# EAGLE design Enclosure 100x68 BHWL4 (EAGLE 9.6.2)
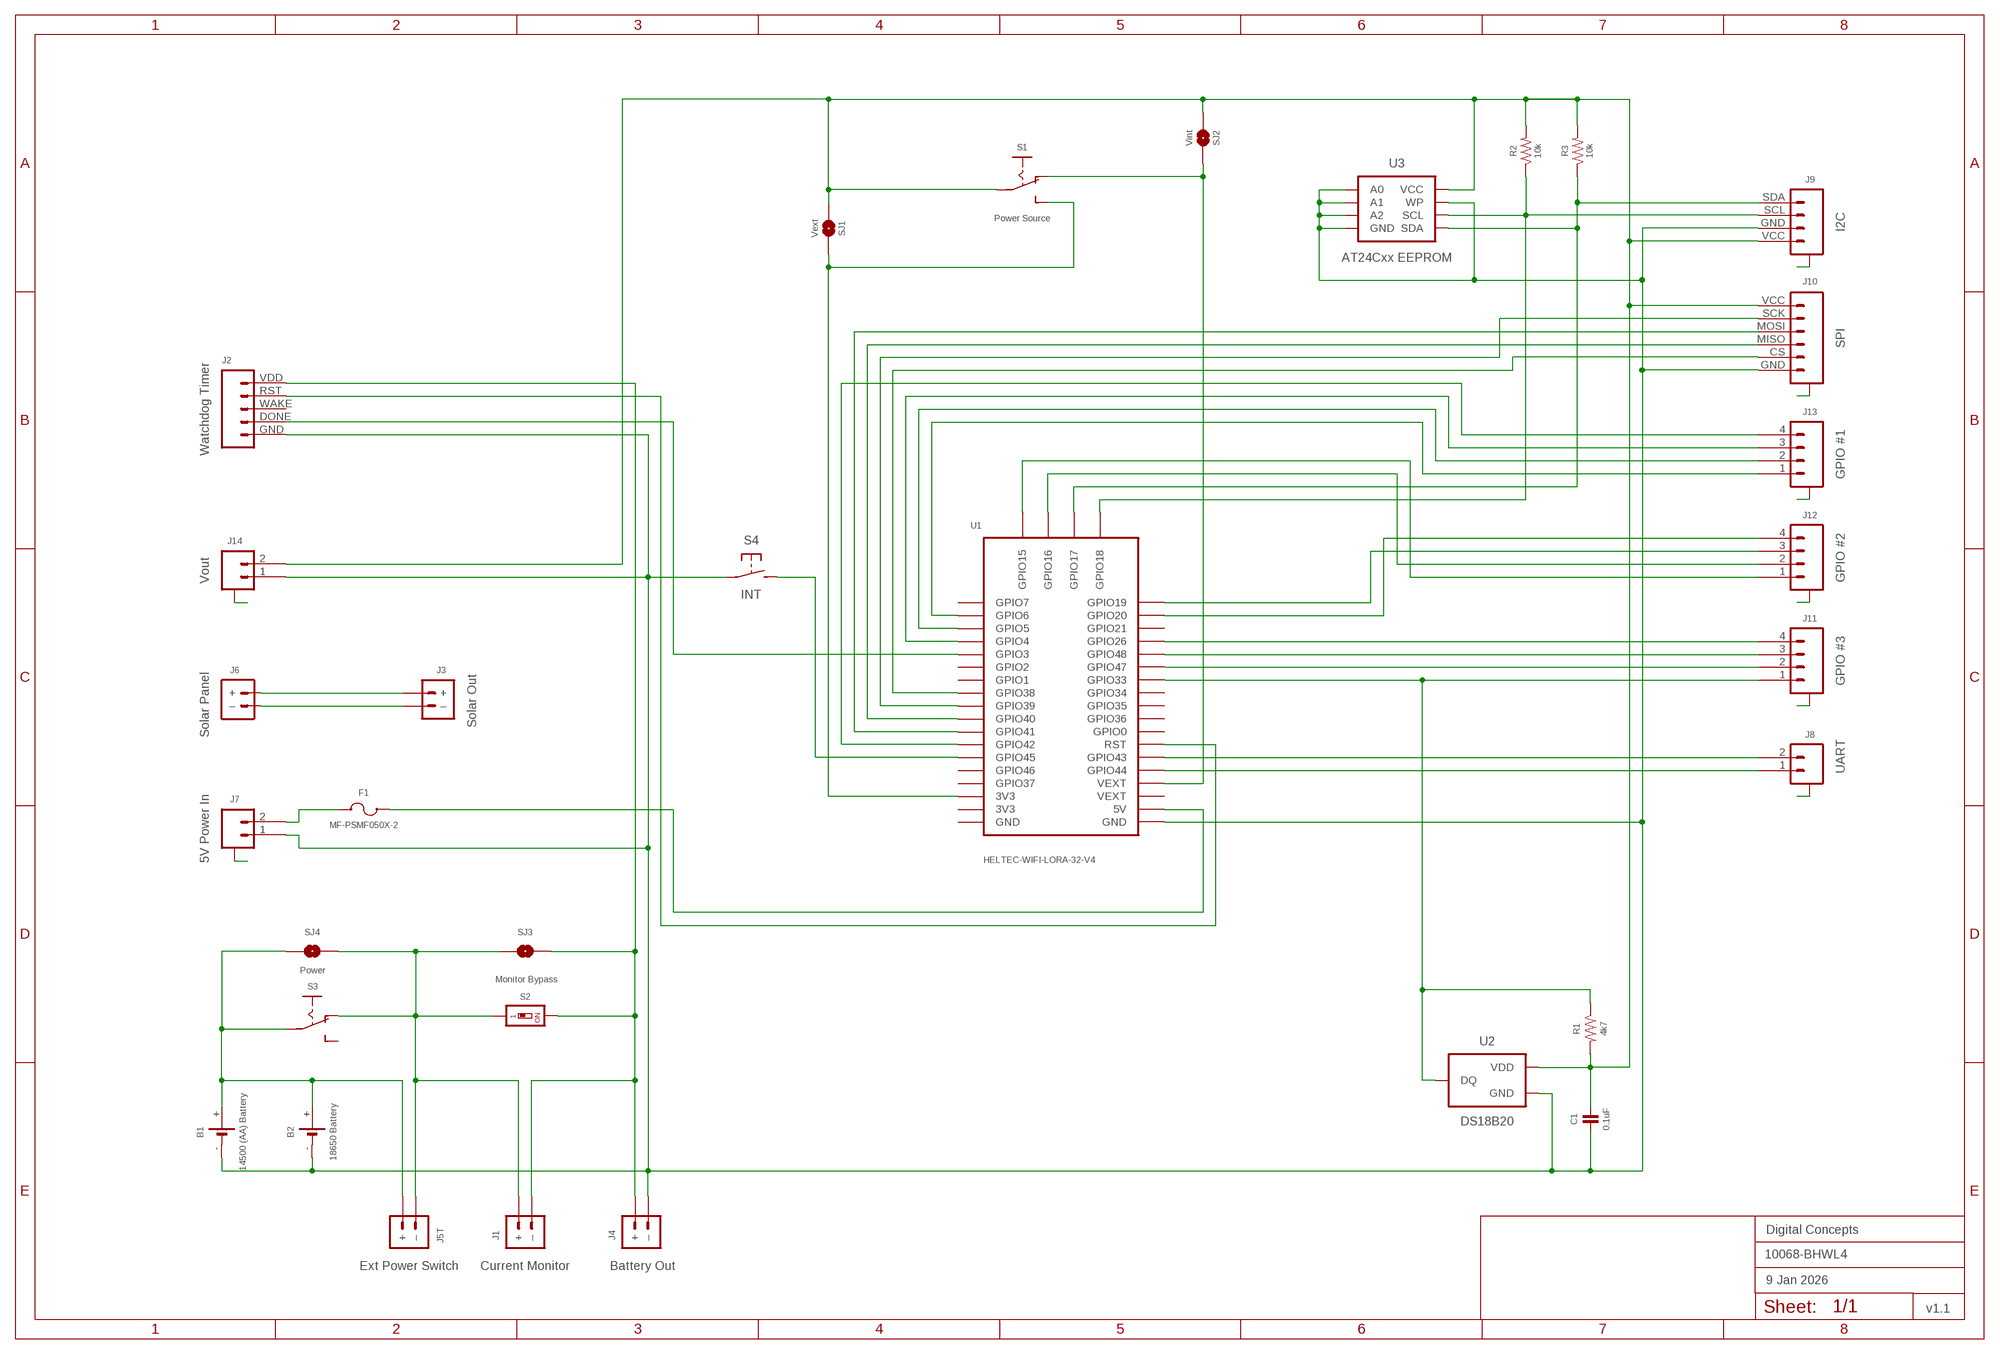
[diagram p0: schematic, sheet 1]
FRAME2 (A3L-LOC): DATE: 9 Jan 2026; OWNER: Digital Concepts; TITLE: 10068-BHWL4; VERSION: v1.1

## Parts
B1  14500 (AA) Battery  BATTERY-HOLDER-14500(AA)  [BATTERY-14500]
B2  18650 Battery  BATTERY-HOLDER-18650  [BATTERY-18650]
C1  0.1uF  CAPACITOR-0805  [C0805]
F1  MF-PSMF050X-2  [F0805]
J1  Current Monitor  JST-PH2.0-2-HORIZONTALJST-PTH-2  [JST-PH2.0-2-HORIZONTAL]
J2  Watchdog Timer  HEADER-1X5-WDT  [CONN_05-WDT]
J3  Solar Out  JST-GH1.25-2-HORIZONTAL-POWER  [JST-GH1.25-2-HORIZONTAL]
J4  Battery Out  JST-GH1.25-2-HORIZONTAL-POWER  [JST-GH1.25-2-HORIZONTAL]
J5T  Ext Power Switch  JST-PH2.0-2-DUAL-POWERJST-PTH-2  [JST-PH2.0-2-DUAL-POWER]
J6  Solar Panel  JST-PH2.0-2-VERTICAL  [JST-PH2.0-2-VERTICAL=POWER]
J7  5V Power In  JST-SH1.0-2-SMD-HORIZONTAL  [JST-SH1.0-2-SMD-HORIZONTAL]
J8  UART  JST-SH1.0-2-SMD-HORIZONTAL  [JST-SH1.0-2-SMD-HORIZONTAL]
J9  I2C  JST-SH1.0-4-SMD-HORIZONTAL-I2C  [JST-SH1.0-4-SMD-HORIZONTAL-I2C]
J10  SPI  JST-SH1.0-6-SMD-HORIZONTAL-SPI  [JST-SH1.0-6-SMD-HORIZONTAL-SPI]
J11  GPIO #3  JST-SH1.0-4-SMD-HORIZONTAL  [JST-SH1.0-4-SMD-HORIZONTAL]
J12  GPIO #2  JST-SH1.0-4-SMD-HORIZONTAL  [JST-SH1.0-4-SMD-HORIZONTAL]
J13  GPIO #1  JST-SH1.0-4-SMD-HORIZONTAL  [JST-SH1.0-4-SMD-HORIZONTAL]
J14  Vout  JST-SH1.0-2-SMD-HORIZONTAL  [JST-SH1.0-2-SMD-HORIZONTAL]
R1  4k7  RESISTORR0805  [R0805]
R2  10k  RESISTORR0805  [R0805]
R3  10k  RESISTORR0805  [R0805]
S1  Power Source  SWITCH-SLIDE-SPDT-SMT  [SWITCH-SPDT-SMT]
S2  Monitor Bypass  SWITCH-DIP-SWS001  [SMD-001]
S3  Power  SWITCH-SLIDE-SPDT-PTH  [SWITCH-SPDT-PTH]
S4  INT  SWITCH-MOMENTARY-2-PIN  [SWITCH-2-PAD]
SJ1  Vext  SJ  [SJ]
SJ2  Vint  SJ-V-2  [SJ-VIA-2]
SJ3  Monitor  SJ  [SJ]
SJ4  Power  SJ  [SJ]
U1  HELTEC-WIFI-LORA-32-V4  [HELTEC-WIFI-LORA-32-V4]
U2  DS18B20  THERMOMETER-DS18B20  [TO-92]
U3  AT24Cxx EEPROM  AT24CXX-EEPROM  [SOP-8]

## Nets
3V3: S1.3(S) SJ1.1 U1.3V3@38(3V3)
5V: F1.1 U1.5V
A2: J11.A@1(A) J11.A@4(A)
A3: J12.A@1(A) J12.A@4(A)
A4: J10.A@1(A) J10.A@6(A)
A5: J14.A@1(A) J14.A@2(A)
A6: J8.A@1(A) J8.A@2(A)
A7: J9.A@1(A) J9.A@4(A)
A8: J13.A@1(A) J13.A@4(A)
A13: J7.A@1(A) J7.A@2(A)
BAT+: B1.+ B2.+ J5T.+ S3.2(P) SJ4.2
CS: J10.CS U1.GPIO38
GND: B1.- B2.- C1.2 J2.GND J4.-(–) J7.1 J9.GND J10.GND J14.1 S4.P$1(P) U1.GND@1(GND) U2.1(GND) U3.P$1(A0) U3.P$2(A1) U3.P$3(A2) U3.P$4(GND) U3.P$7(WP)
GPIO3: J2.DONE U1.GPIO3
GPIO4: J13.3 U1.GPIO4
GPIO5: J13.2 U1.GPIO5
GPIO6: J13.1 U1.GPIO6
GPIO15: J12.1 U1.GPIO15
GPIO16: J12.2 U1.GPIO16
GPIO19: J12.3 U1.GPIO19
GPIO20: J12.4 U1.GPIO20
GPIO26: J11.4 U1.GPIO26
GPIO33: J11.1 R1.1 U1.GPIO33 U2.2(DQ)
GPIO42: J13.4 U1.GPIO42
GPIO45: S4.P$2(S) U1.GPIO45
GPIO47: J11.2 U1.GPIO47
GPIO48: J11.3 U1.GPIO48
MCU-BAT+: J1.2(–) J2.VDD J4.+ S2.2 SJ3.1
MISO: J10.MISO U1.GPIO40
MOSI: J10.MOSI U1.GPIO41
N$14: F1.2 J7.2
POWER+: J1.1(+) J5T.-(–) S2.1 S3.1(O) SJ3.2 SJ4.1
RST: J2.RST U1.RST
RX: J8.1 U1.GPIO44
SCK: J10.SCK U1.GPIO39
SCL: J9.SCL R2.1 U1.GPIO18 U3.P$6(SCL)
SDA: J9.SDA R3.1 U1.GPIO17 U3.P$5(SDA)
SOLAR+: J3.+ J6.+
SOLAR-: J3.-(–) J6.-(–)
TX: J8.2 U1.GPIO43
VCC: C1.1 J9.VCC J10.VCC J14.2 R1.2 R2.2 R3.2 S1.2(P) SJ1.2 SJ2.2 SJ2.2@V U2.3(VDD) U3.P$8(VCC)
VEXT: S1.1(O) SJ2.1 U1.VEXT@4(VEXT)
Unconnected: J2.WAKE S3.3(S) U1.3V3@39(3V3) U1.GND@40(GND) U1.GPIO0 U1.GPIO1 U1.GPIO2 U1.GPIO7 U1.GPIO21 U1.GPIO34 U1.GPIO35 U1.GPIO36 U1.GPIO37 U1.GPIO46 U1.VEXT@3(VEXT)

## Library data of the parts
B1 = digitalconcepts:BATTERY-HOLDER-14500(AA): 14500 (AA) battery holder
B2 = digitalconcepts:BATTERY-HOLDER-18650: 18650 Battery Holder
C1 = digitalconcepts:CAPACITOR-0805: 0805 Capacitor
F1 = digitalconcepts:MF-PSMF050X-2: PTC Resettable Fuse
J1 = digitalconcepts:JST-PH2.0-2-HORIZONTAL: PH2.0 2P Right Angle PCB Connector; PROD_ID: CONN-09863; SKU: PRT-09914
J2 = digitalconcepts:HEADER-1X5-WDT: Single Row 5-Pin Header
J3 J4 = digitalconcepts:JST-GH1.25-2-HORIZONTAL-POWER: JST GH1.25 2P PTH Connector (Power)
J5T = digitalconcepts:JST-PH2.0-2-DUAL-POWER: JST PH2.0 2P PTH Dual-Side Connector (Power); PROD_ID: CONN-09863; SKU: PRT-09914
J6 = digitalconcepts:JST-PH2.0-2-VERTICAL: PH2.0 2P PCB Connector
J7 J8 J14 = digitalconcepts:JST-SH1.0-2-SMD-HORIZONTAL: JST SH1.0 2P SMD Horizontal Connector
J9 = digitalconcepts:JST-SH1.0-4-SMD-HORIZONTAL-I2C: JST SH1.0 4P SMD I2C horizontal connector
J10 = digitalconcepts:JST-SH1.0-6-SMD-HORIZONTAL-SPI: JST SH1.0 6P SMD SPI horizontal connector
J11-J13 = digitalconcepts:JST-SH1.0-4-SMD-HORIZONTAL: JST SH1.0 4P SMD horizontal connector
R1-R3 = digitalconcepts:RESISTOR: Resistor; SPICEPREFIX: R
S1 = digitalconcepts:SWITCH-SLIDE-SPDT-SMT: Mini Sliding Switch SPDT SMT
S2 = digitalconcepts:SWITCH-DIP-SWS001: SMD Dip Switch 1 pol.
S3 = digitalconcepts:SWITCH-SLIDE-SPDT-PTH: Mini Sliding Switch SPDT PTH
S4 = digitalconcepts:SWITCH-MOMENTARY-2-PIN: 2 Pin Momentary Switch
SJ1 SJ3 SJ4 = digitalconcepts:SJ: Solder Jumper
SJ2 = digitalconcepts:SJ-V-2: Solder Jumper with Pad Vias
U1 = digitalconcepts:HELTEC-WIFI-LORA-32-V4: Heltec WiFi LoRa 32 Development Board V4
U2 = digitalconcepts:THERMOMETER-DS18B20: Digital Thermometer -55C-125C TO92-3; AVAILABILITY: Bad; DESCRIPTION: Temperature Sensor Digital, Local -55°C ~ 125°C 12 b 8-uMAX; MF: Maxim Integrated; MP: DS18B20; PACKAGE: TO-92 Maxim Integrated; PRICE: None
U3 = digitalconcepts:AT24CXX-EEPROM: AT24Cxx EEPROM SOP-8

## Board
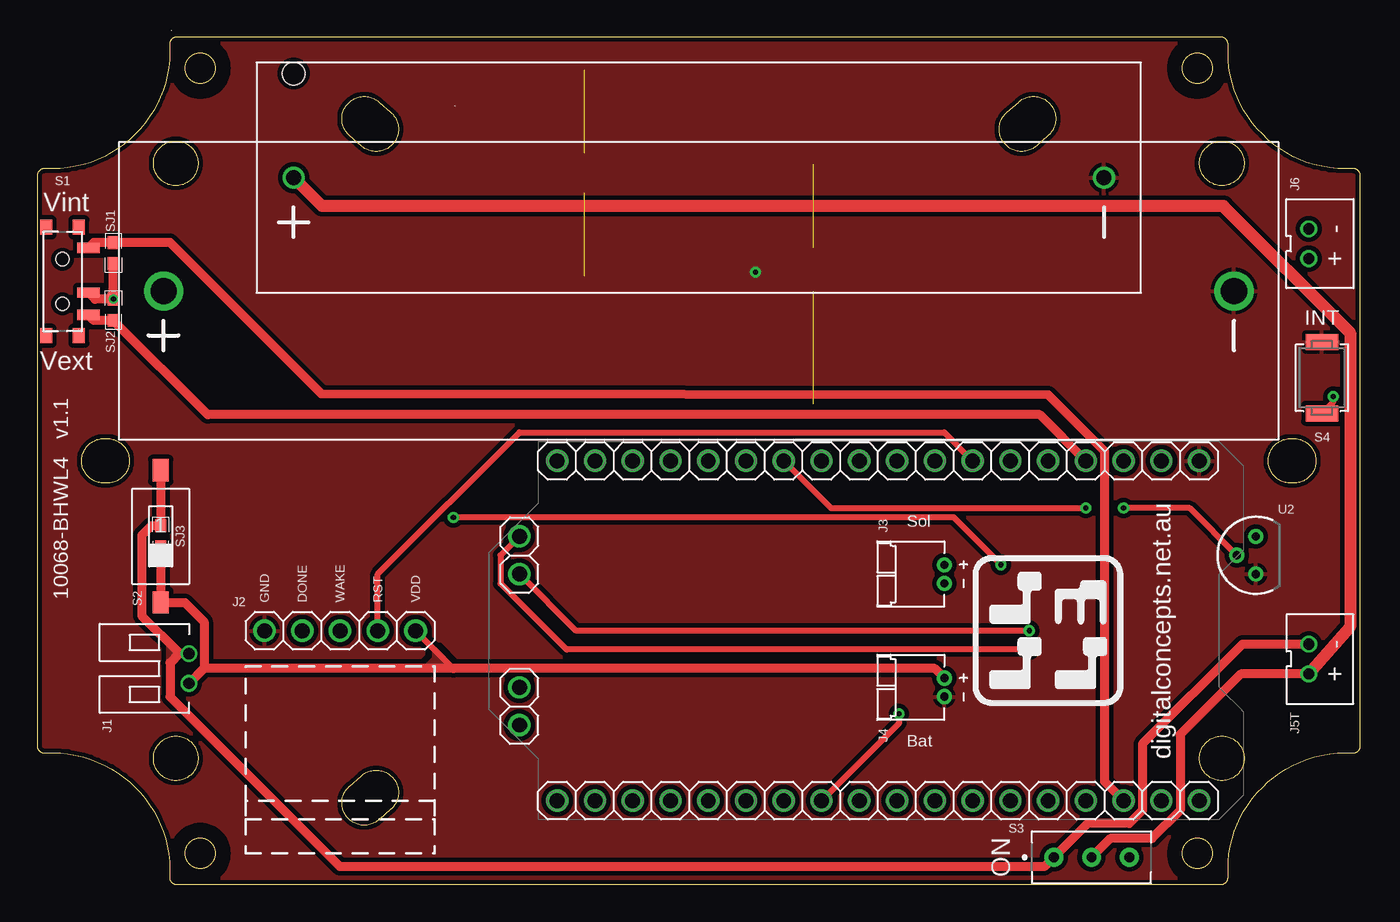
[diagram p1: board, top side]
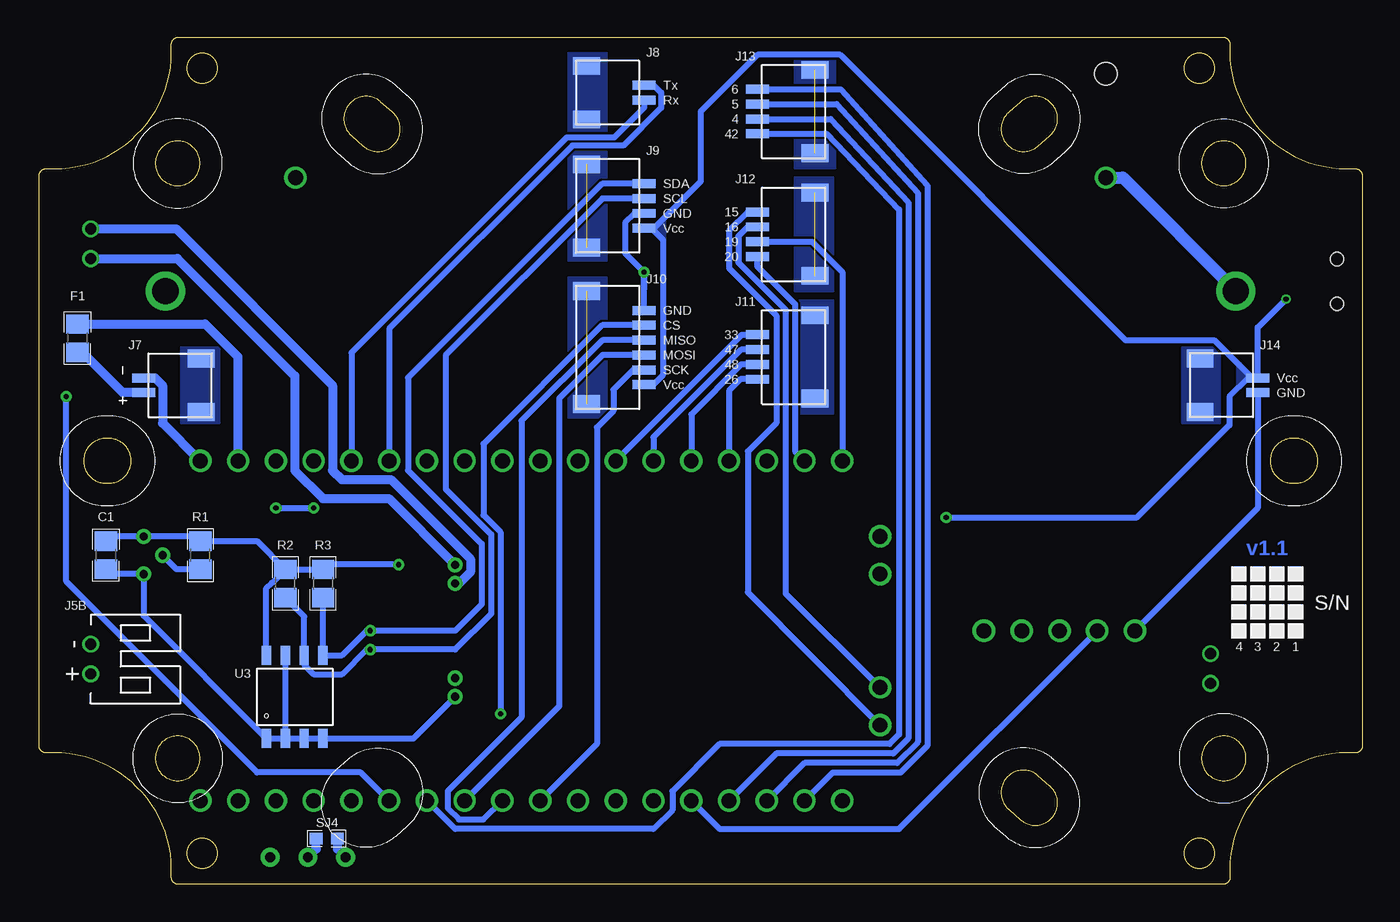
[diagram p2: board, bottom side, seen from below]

Size 89 x 57 mm. Coordinates in mm from the lower left corner, seen from the top.
Outline: 1134 segments
Outline: circle at 10.97,2.08 radius 1.02
Outline: circle at 10.97,54.92 radius 1.02
Outline: circle at 78.03,54.92 radius 1.02
Outline: circle at 78.03,2.08 radius 1.02
Copper layers (1*16): Top 0.035mm / dielectric 1.5mm / Bottom 0.035mm
Design rules "default *": minimum track width 6mil, minimum drill 0.35mm, track to track 6mil, track to pad 6mil, pad to pad 6mil, via to via 6mil, smd to smd 6mil, copper to edge 6mil, drill to drill 6mil, minimum pad ring 1mil, minimum via ring 8mil, stop-mask expansion 4mil, vias tented up to drill 0mil, thermal gap 10mil

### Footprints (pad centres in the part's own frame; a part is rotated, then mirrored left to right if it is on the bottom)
BATTERY-14500 = drill 1: + -27.25,0; - 27.25,0 | hole 1.524: -27.25,7
BATTERY-18650 = drill 1.75: + -36,0; - 36,0
C0805 = smd 1.3 x 1.5: 1 -0.95,0; 2 0.95,0
F0805 = smd 1.3 x 1.5: 1 -0.95,0; 2 0.95,0
JST-PH2.0-2-HORIZONTAL = drill 0.75: 1 1,0; 2 -1,0
CONN_05-WDT = drill 1 pad 1.524: DONE 2.54,0; GND 0,0; RST 7.62,0; VDD 10.16,0; WAKE 5.08,0
JST-GH1.25-2-HORIZONTAL = drill 0.55 pad 1.016: + -0.625,0; - 0.625,0
JST-PH2.0-2-DUAL-POWER = drill 0.75: + 1,0; - -1,0
JST-PH2.0-2-VERTICAL=POWER = drill 0.75: + -1,0; - 1,0
JST-SH1.0-2-SMD-HORIZONTAL = smd 0.6 x 1.55: 1 0.5,2.54; 2 -0.5,2.54 | smd 1.2 x 1.8: A@1 1.8,-1.335; A@2 -1.8,-1.335
JST-SH1.0-4-SMD-HORIZONTAL-I2C = smd 1.2 x 1.8: A@1 2.8,-1.335; A@4 -2.8,-1.335 | smd 0.6 x 1.55: GND 0.5,2.54; SCL -0.5,2.54; SDA -1.5,2.54; VCC 1.5,2.54
JST-SH1.0-6-SMD-HORIZONTAL-SPI = smd 1.2 x 1.8: A@1 3.8,-1.335; A@6 -3.8,-1.335 | smd 0.6 x 1.55: CS -1.5,2.54; GND -2.5,2.54; MISO -0.5,2.54; MOSI 0.5,2.54; SCK 1.5,2.54; VCC 2.5,2.54
JST-SH1.0-4-SMD-HORIZONTAL = smd 0.6 x 1.55: 1 1.5,2.54; 2 0.5,2.54; 3 -0.5,2.54; 4 -1.5,2.54 | smd 1.2 x 1.8: A@1 2.8,-1.335; A@4 -2.8,-1.335
R0805 = smd 1.3 x 1.5: 1 -0.95,0; 2 0.95,0
SWITCH-SPDT-SMT = smd 0.7 x 1.5: 1 2.25,1.75; 2 0.75,1.75; 3 -2.25,1.75 | smd 1 x 0.8: GND@1 3.65,-1.1; GND@2 3.65,1.1; GND@3 -3.65,1.1; GND@4 -3.65,-1.1 | hole 0.9: -1.5,0; 1.5,0
SMD-001 = smd 1.1 x 1.5: 1 0,-4.45; 2 0,4.45
SWITCH-SPDT-PTH = drill 0.65 pad 1.27: 1 -2.54,0; 2 0,0; 3 2.54,0
SWITCH-2-PAD = smd 1.067 x 2.184: P$1 -2.4,0; P$2 2.4,0
SJ = smd 0.864 x 0.762: 1 -0.711,0; 2 0.711,0
SJ-VIA-2 = smd 0.864 x 0.762: 1 -0.711,0; 2 0.711,0 | drill 0.35 pad 0.61: 2@V 0.711,0
HELTEC-WIFI-LORA-32-V4 = drill 1: 3V3@38 -22.86,5.08; 3V3@39 -22.86,2.54; 5V 0,2.54; GND@1 0,0; GND@40 -22.86,0; GPIO0 0,17.78; GPIO1 -22.86,27.94; GPIO2 -22.86,30.48; GPIO3 -22.86,33.02; GPIO4 -22.86,35.56; GPIO5 -22.86,38.1; GPIO6 -22.86,40.64; GPIO7 -22.86,43.18; GPIO15 -17.78,45.72; GPIO16 -15.24,45.72; GPIO17 -7.62,45.72; GPIO18 -5.08,45.72; GPIO19 0,43.18; GPIO20 0,40.64; GPIO21 0,38.1; GPIO26 0,35.56; GPIO33 0,27.94; GPIO34 0,25.4; GPIO35 0,22.86; GPIO36 0,20.32; GPIO37 -22.86,7.62; GPIO38 -22.86,25.4; GPIO39 -22.86,22.86; GPIO40 -22.86,20.32; GPIO41 -22.86,17.78; GPIO42 -22.86,15.24; GPIO43 0,12.7; GPIO44 0,10.16; GPIO45 -22.86,12.7; GPIO46 -22.86,10.16; GPIO47 0,30.48; GPIO48 0,33.02; RST 0,15.24; VEXT@3 0,5.08; VEXT@4 0,7.62
TO-92 = drill 0.55 pad 1.016: 1 -1.27,0; 2 0,1.27; 3 1.27,0
SOP-8 = smd 0.635 x 1.27: P$1 -1.905,-2.794; P$2 -0.635,-2.794; P$3 0.635,-2.794; P$4 1.905,-2.794; P$5 1.905,2.794; P$6 0.635,2.794; P$7 -0.635,2.794; P$8 -1.905,2.794

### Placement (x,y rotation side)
B1  44.5,47.55 0 top
B2  44.5,39.93 0 top
C1  84.5,22.15 270 bottom
F1  86.41,36.75 270 bottom
J1  10.21,14.53 90 top
J2  15.29,17.07 0 top
J3  61.01,20.88 270 top
J4  61.01,13.26 270 top
J5T  85.52,15.16 270 bottom
J6  85.52,43.1 90 top
J7  79.42,33.58 90 bottom
J8  50.85,53.26 270 bottom
J9  50.85,45.64 270 bottom
J10  50.85,36.12 270 bottom
J11  38.15,35.48 90 bottom
J12  38.15,43.74 90 bottom
J13  38.15,51.99 90 bottom
J14  9.57,33.58 270 bottom
R1  78.15,22.15 90 bottom
R2  72.44,20.24 90 bottom
R3  69.9,20.24 90 bottom
S1  1.7,40.56 270 top
S2  8.3,23.42 180 top
S3  70.92,1.83 0 top
S4  86.41,34.09 270 top
SJ1  5.13,42.47 270 top
SJ2  5.13,38.66 90 top
SJ3  8.3,23.42 90 top
SJ4  69.65,3.1 180 bottom
U1  78.15,28.5 90 top
U2  81.96,22.15 90 top
U3  71.8,12.62 0 bottom

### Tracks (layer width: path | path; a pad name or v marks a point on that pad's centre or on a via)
3V3
  Top 0.61: S1.3 3.82,43.18 SJ1.1 8.94,43.18 19.12,33 68,32.94 71.8,29.13 71.8,6.91 U1.3V3@38
5V
  Bottom 0.61: F1.1 77.83,37.7 75.61,35.48 U1.5V
$X
  cutout Bottom: 10.97,56.95 arc180 10.97,52.88 arc180
$X1
  cutout Bottom: 78.03,56.95 arc180 78.03,52.88 arc180
$X2
  cutout Top: 78.03,4.12 arc180 78.03,0.05 arc180
$X3
  cutout Top: 10.97,4.12 arc180 10.97,0.05 arc180
$X4
  cutout Top: 10.97,56.95 arc180 10.97,52.88 arc180
$X5
  cutout Top: 78.03,56.95 arc180 78.03,52.88 arc180
$X6
  cutout Bottom: 78.03,4.12 arc180 78.03,0.05 arc180
$X7
  cutout Bottom: 10.97,4.12 arc180 10.97,0.05 arc180
A2
  pour Bottom (no thermals): 35.61,39.29 38.15,39.29 38.15,31.67 35.61,31.67
A3  (1 unrouted)
  pour Bottom (no thermals): 35.61,47.55 38.15,47.55 38.15,39.93 35.61,39.93
A4  (1 unrouted)
  pour Bottom (no thermals): 50.85,31.42 53.39,31.42 53.39,40.82 50.85,40.82
A5
  pour Bottom (no thermals): 9.57,36.12 12.11,36.12 12.11,31.04 9.57,31.04
A6
  pour Bottom (no thermals): 53.39,55.93 53.39,50.6 50.85,50.6 50.85,55.93
A7  (1 unrouted)
  pour Bottom (no thermals): 50.85,49.33 53.39,49.33 53.39,41.96 50.85,41.96
A8  (1 unrouted)
  pour Bottom (no thermals): 35.48,55.8 38.15,55.8 38.15,48.18 35.48,48.18
A13
  pour Bottom (no thermals): 79.42,36.12 76.88,36.12 76.88,31.04 79.42,31.04
BAT+
  Top 0.61: J5T.+ 80.96,14.16 76.88,10.08 76.88,5 74.98,3.1 72.19,3.1 S3.2
  Top 0.813: B1.+ 19.15,45.64 79.79,45.64 88.31,37.12 88.31,17.34 J5T.+
  Bottom 0.61: S3.2 70.36,2.39 SJ4.2
  Bottom 0.813: B1.+ 16.12,47.55 B2.+
CS  (via drill 0.35)
  Top 0.406: v57.96,11.48 57.96,10.85 U1.GPIO38
  Bottom 0.406: J10.CS 51.13,37.62 59.1,29.64 59.1,24.84 57.96,23.7 v57.96,11.48
GND  (via drill 0.35)
  Bottom 0.406: U3.P$7 U3.P$2 | U3.P$2 U3.P$1 81.96,18.09 U2.1 84.42,20.88 C1.2 | U3.P$2 U3.P$3 U3.P$4 63.81,9.83 J4.- | J10.GND v48.31,41.2 | v48.31,41.2 48.31,40.06 | J9.GND 48.94,45.14 49.58,44.51 49.58,42.47 v48.31,41.2 | J2.GND 7.03,25.32 J14.1
  Bottom 0.61: U1.GND@1 80.69,31.04 80.69,33.57 81.2,34.08 J7.1
  pour Top (isolate 0.305, rank 2): -1.65,58.87 -1.65,-1.92 90.59,-1.92 90.59,58.87
GPIO3
  Bottom 0.406: J2.DONE 31.16,3.73 43.23,3.73 U1.GPIO3
GPIO4
  Bottom 0.406: J13.3 35.74,51.49 30.53,45.9 30.53,9.83 31.55,8.81 39.42,8.81 U1.GPIO4
GPIO5
  Bottom 0.406: J13.2 35.35,52.49 29.89,46.53 29.89,9.58 31.29,8.18 37.51,8.18 U1.GPIO5
GPIO6
  Bottom 0.406: J13.1 35.08,53.49 29.26,47.04 29.26,9.32 31.04,7.54 35.61,7.54 U1.GPIO6
GPIO15
  Bottom 0.406: U1.GPIO15 41.32,19.65 41.32,29.13 39.42,31.04 39.42,38.28 42.59,41.45 42.59,43.97 41.32,45.24 J12.1
GPIO16
  Bottom 0.406: U1.GPIO16 38.78,19.57 38.78,38.66 41.96,41.83 41.96,43.6 41.32,44.24 J12.2
GPIO19
  Bottom 0.406: U1.GPIO19 34.97,41.21 37.01,43.24 J12.3
GPIO20
  Bottom 0.406: U1.GPIO20 38.15,29.13 38.15,39.04 40.69,41.58 J12.4
GPIO26
  Bottom 0.406: J11.4 41.83,33.98 42.59,33.22 U1.GPIO26
GPIO33  (via drill 0.35)
  Top 0.406: v73.07,25.32 77.52,25.32 U2.2 | U1.GPIO33 53.39,25.32 v70.53,25.32
  Bottom 0.406: R1.1 79.74,21.2 U2.2 | v73.07,25.32 v70.53,25.32 | J11.1 41.73,36.98 U1.GPIO33
GPIO42
  Bottom 0.406: J13.4 36.01,50.49 31.16,45.4 31.16,10.08 31.8,9.45 43.23,9.45 46.4,6.27 46.4,5 47.67,3.73 61.01,3.73 U1.GPIO42
GPIO45  (via drill 0.35)
  Top 0.406: v87.17,32.82 87.17,32.45 S4.P$2
  Bottom 0.406: U1.GPIO45 67.36,7.54 74.34,7.54 87.17,20.37 v87.17,32.82
GPIO47
  Bottom 0.406: J11.2 41.78,35.98 47.67,30.09 U1.GPIO47
GPIO48
  Bottom 0.406: J11.3 41.78,34.98 45.13,31.63 U1.GPIO48
MCU-BAT+
  Top 0.406: J2.VDD 27.99,14.53
  Top 0.61: SJ3.1 S2.2 9.93,18.97 11.19,17.7 11.23,17.67 11.23,14.55 J1.2 11.21,14.53 27.99,14.53 60.36,14.53 J4.+
  pour Top (no thermals): 27.99,14.53 26.72,15.8 26.72,15.16 26.08,14.53
MISO
  Bottom 0.406: J10.MISO 51.1,36.62 56.56,31.2 56.56,11.23 61.52,6.27 61.52,5.13 60.76,4.37 59.1,4.37 U1.GPIO40
MOSI
  Bottom 0.406: J10.MOSI 51.1,35.62 54.02,32.69 54.02,11.99 U1.GPIO41
N$14
  Bottom 0.61: J7.2 83.37,33.08 86.09,35.8 F1.2
POWER+
  Top 0.61: S2.1 SJ3.2 7.67,24.13 7.03,23.5 7.03,18.07 9.57,15.53 J1.1 9.55,15.53 8.94,14.92 8.94,12.62 20.37,1.19 67.74,1.19 S3.1 70.66,4.12 73.46,4.12 74.34,5 74.34,9.45 81.06,16.16 J5T.-
  Bottom 0.61: S3.1 68.93,2.39 SJ4.1
  pour Top (no thermals): 9.55,15.55 8.94,16.16 8.94,14.94
RST
  Top 0.406: U1.RST 61.01,30.4 32.43,30.4 22.91,20.88 J2.RST
RX
  Bottom 0.406: U1.GPIO44 67.99,35.77 53.49,50.27 50.3,50.27 48.31,52.26 J8.1
SCK
  Bottom 0.406: J10.SCK 49.05,34.62 50.38,33.29 50.38,31.85 51.48,30.75 51.48,9.45 U1.GPIO39
SCL  (via drill 0.35)
  Top 0.406: v66.72,15.8 35.61,15.8 31.16,20.24 31.16,22.15 U1.GPIO18
  Bottom 0.406: R2.1 71.17,18.02 U3.P$6 71.17,14.78 70.53,14.15 68.63,14.15 66.98,15.8 v66.72,15.8 61.01,15.8 58.6,18.21 58.6,23.55 61.64,26.59 61.64,35.61 51.11,46.14 J9.SCL
SDA  (via drill 0.35)
  Top 0.406: v66.72,17.07 36.24,17.07 U1.GPIO17
  Bottom 0.406: R3.1 U3.P$5 68.63,15.42 66.98,17.07 v66.72,17.07 61.01,17.07 59.23,18.85 59.23,22.91 64.18,27.86 64.18,34.09 51.13,47.14 J9.SDA
SOLAR+
  Bottom 0.61: J3.+ 65.46,25.96 69.9,25.96 71.8,27.86 71.8,34.21 79.69,42.1 J6.+
SOLAR-
  Bottom 0.61: J6.- 79.79,44.1 69.26,33.58 69.26,27.86 68.63,27.23 65.33,27.23 59.99,21.9 59.99,21.02 60.76,20.25 J3.-
TX
  Bottom 0.406: J8.2 47.67,53.76 47.17,53.26 47.17,52.25 49.71,49.71 53.14,49.71 65.45,37.39 U1.GPIO43
VCC  (via drill 0.35)
  Top 0.406: v64.82,21.51 61.64,24.69 v27.99,24.69
  Top 0.61: S1.2 3.89,39.37 SJ2.2@V SJ1.2
  Bottom 0.406: C1.1 84.18,23.42 U2.3 78.47,23.42 R1.2 74.34,23.1 R2.2 | R2.2 73.33,20.3 73.34,20.3 73.71,19.93 U3.P$8 | R2.2 R3.2 69.58,21.51 v64.82,21.51 | J10.VCC 47.67,33.62 47.04,34.25 47.04,43.38 47.8,44.14 J9.VCC 47.65,44.14 44.5,47.3 44.5,51.99 40.69,55.8 35.11,55.8 15.92,36.62 9.96,36.62 7.42,34.08 | SJ2.2@V 7.03,37.47 J14.2 7.42,34.08 | 7.42,34.08 7.67,34.08 8.94,32.81 8.94,30.9 15.15,24.69 v27.99,24.69
  pour Bottom (no thermals): 47.04,43.36 47.74,44.06 47.04,44.76
  pour Bottom (no thermals): 7.54,34.21 8.3,34.98 8.3,33.45
VEXT
  Top 0.61: S1.1 3.82,37.95 SJ2.1 11.48,31.6 67.44,31.6 U1.VEXT@4

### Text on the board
Bottom: v1.1
tPlace: 10068-BHWL4 v1.1 | digitalconcepts.net.au
bPlace: S/N | 1 | 2 | 3 | 4
tNames: Vint | Vext | Sol | GND | DONE | WAKE | RST | VDD | Bat | ON
bNames: Tx | 6 | Rx | 5 | 4 | 42 | SDA | SCL | 15 | GND | 16 | Vcc | 19 | 20 | GND | 33 | CS | 47 | MISO | 48 | MOSI | Vcc | 26 | SCK | GND | Vcc | J5B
